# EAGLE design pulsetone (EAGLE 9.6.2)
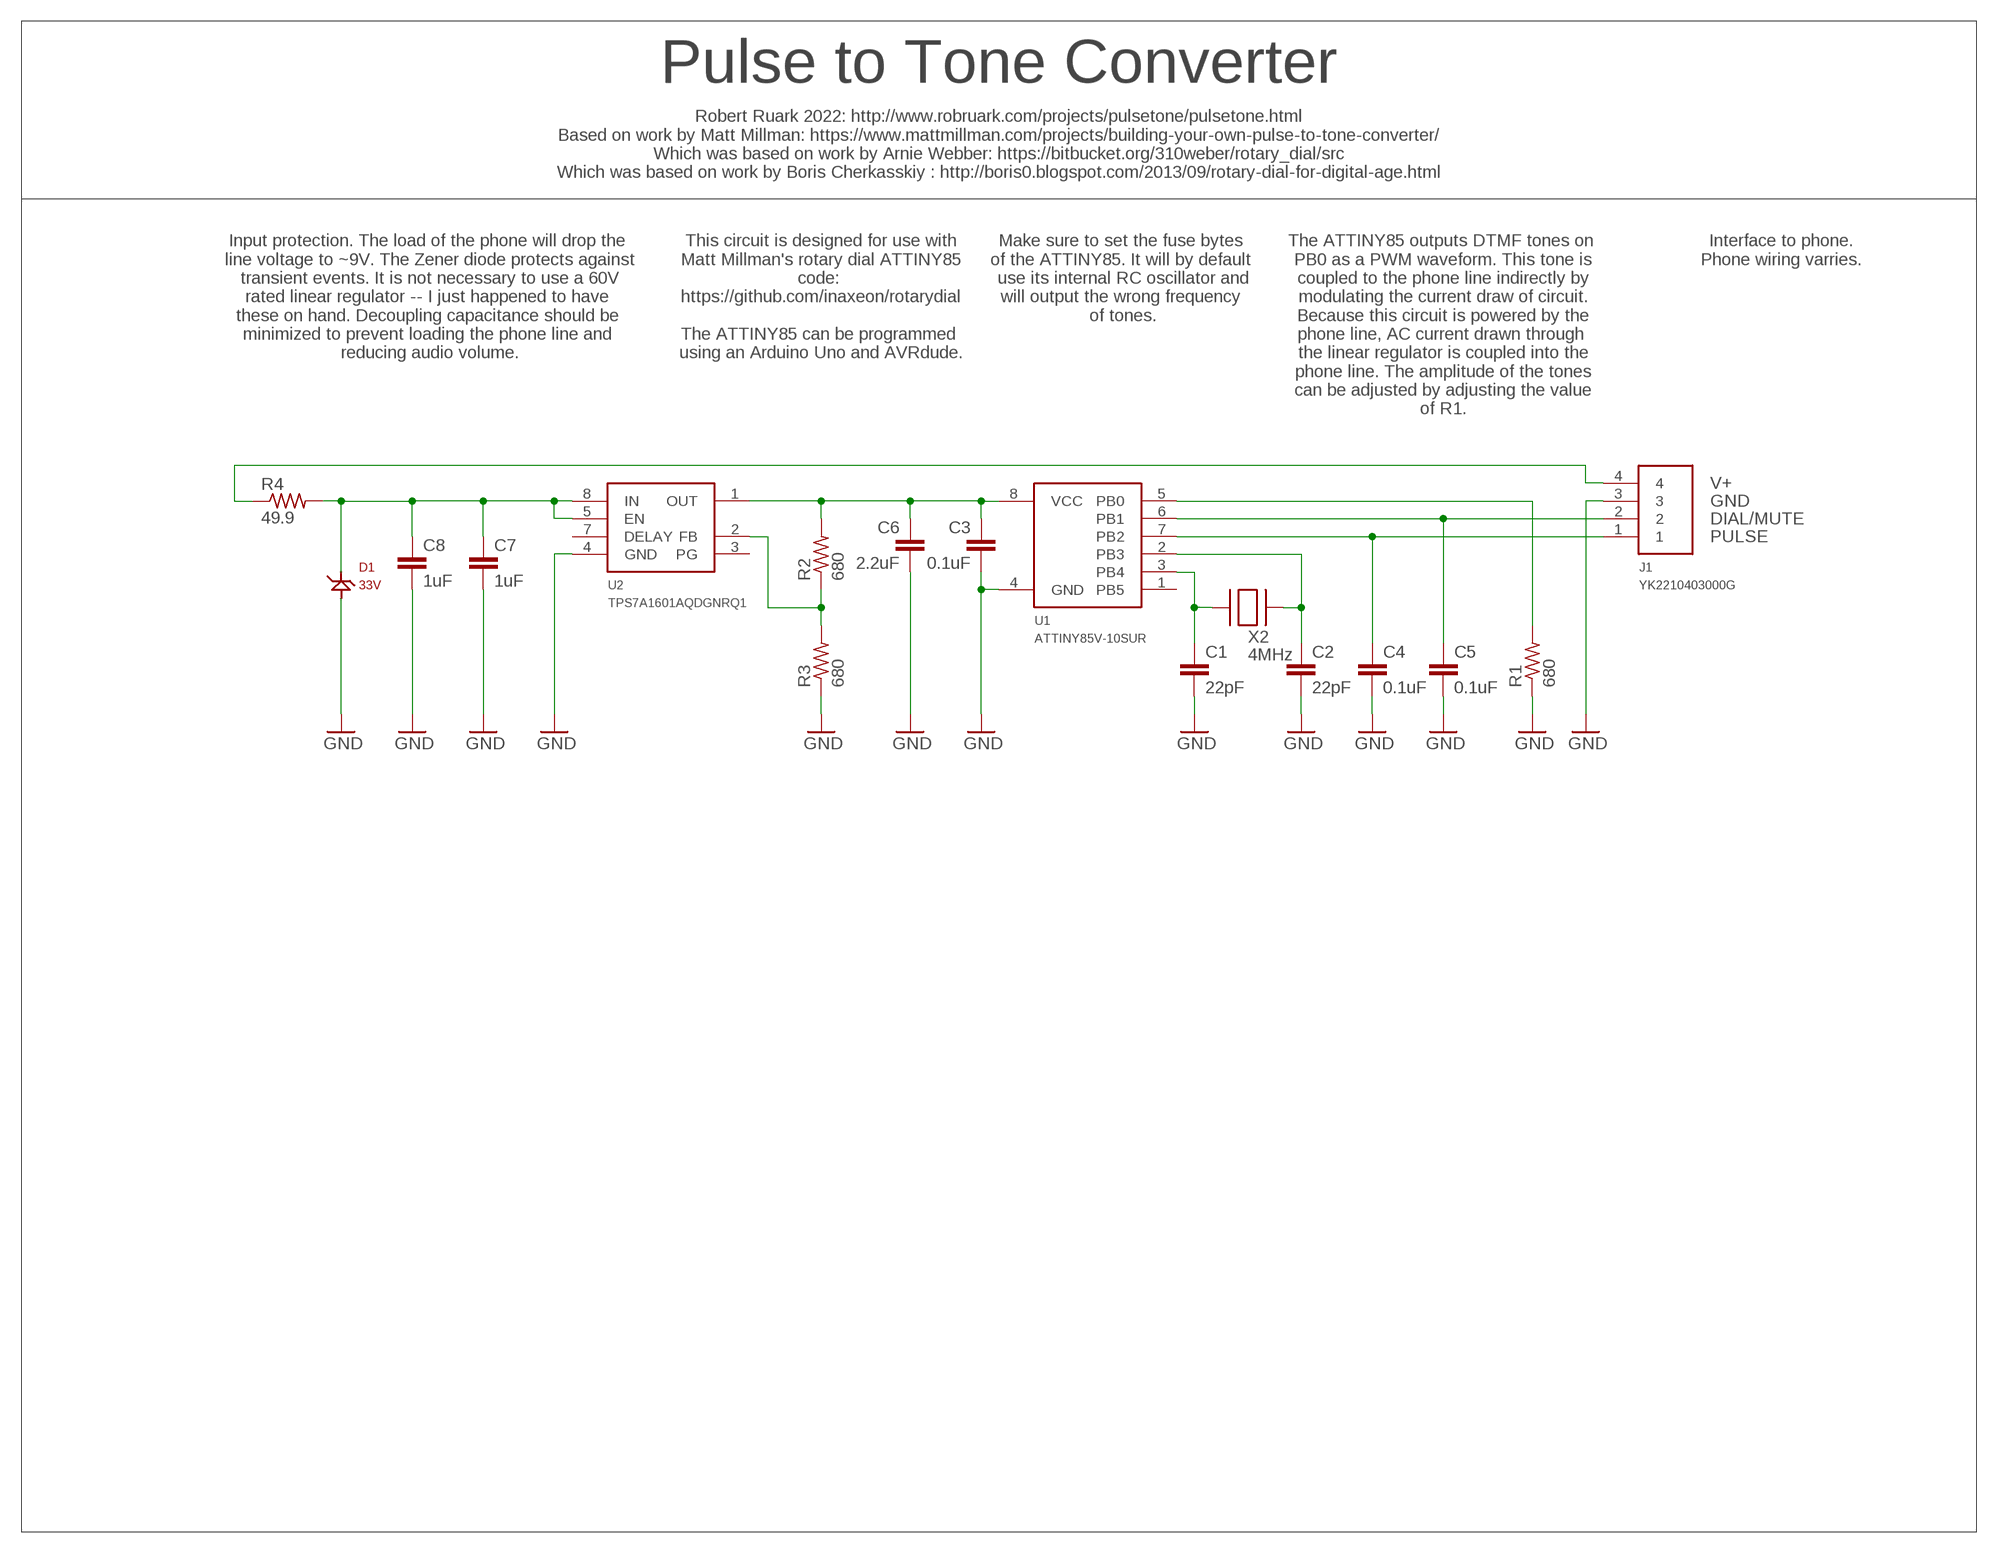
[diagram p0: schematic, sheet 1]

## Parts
C1  22pF  0603_CAPACITOR  [0603]
C2  22pF  0603_CAPACITOR  [0603]
C3  0.1uF  0603_CAPACITOR  [0603]
C4  0.1uF  0603_CAPACITOR  [0603]
C5  0.1uF  0603_CAPACITOR  [0603]
C6  2.2uF  0805_CAPACITOR  [0805]
C7  1uF  1206_CAPACITOR  [1206]
C8  1uF  1206_CAPACITOR  [1206]
D1  33V  1SMA5937BT3GDO-  [DO-214AC]
J1  YK2210403000G  [YK2210403000G]
R1  680  0603_RESISTOR  [0603]
R2  680  0603_RESISTOR  [0603]
R3  680  0603_RESISTOR  [0603]
R4  49.9  1206_RESISTOR  [1206]
U1  ATTINY85V-10SUR  [SOIC8]
U2  TPS7A1601AQDGNRQ1  [MSOP-8]
X2  4MHz  ABLS-4.000MHZ-B2-T  [HC-49/US]

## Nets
GND: C1.2 C2.2 C3.2 C4.2 C5.2 C6.2 C7.2 C8.2 D1.A J1.3 R1.1 R3.1 U1.4(GND) U2.4(GND)
N$1: C1.1 U1.3(PB4) X2.P$1
N$2: C2.1 U1.2(PB3) X2.P$2
N$3: C4.1 J1.1 U1.7(PB2)
N$4: C5.1 J1.2 U1.6(PB1)
N$5: R1.2 U1.5(PB0)
N$7: J1.4 R4.1
N$8: R2.1 R3.2 U2.2(FB)
N$10: C7.1 C8.1 D1.C(K) R4.2 U2.5(EN) U2.8(IN)
VCC: C3.1 C6.1 R2.2 U1.8(VCC) U2.1(OUT)
Unconnected: U1.1(PB5) U2.3(PG) U2.7(DELAY)

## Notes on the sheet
- Pulse to Tone Converter
- Robert Ruark 2022: http://www.robruark.com/projects/pulsetone/pulsetone.html
  Based on work by Matt Millman: https://www.mattmillman.com/projects/building-your-own-pulse-to-tone-converter/
  Which was based on work by Arnie Webber: https://bitbucket.org/310weber/rotary_dial/src
  Which was based on work by Boris Cherkasskiy : http://boris0.blogspot.com/2013/09/rotary-dial-for-digital-age.html
- Input protection. The load of the phone will drop the 
  line voltage to ~9V. The Zener diode protects against
  transient events. It is not necessary to use a 60V
  rated linear regulator -- I just happened to have 
  these on hand. Decoupling capacitance should be 
  minimized to prevent loading the phone line and 
  reducing audio volume.
- This circuit is designed for use with
  Matt Millman's rotary dial ATTINY85
  code: 
  https://github.com/inaxeon/rotarydial
  
  The ATTINY85 can be programmed 
  using an Arduino Uno and AVRdude.
- Make sure to set the fuse bytes 
  of the ATTINY85. It will by default 
  use its internal RC oscillator and
  will output the wrong frequency 
  of tones.
- The ATTINY85 outputs DTMF tones on 
  PB0 as a PWM waveform. This tone is
  coupled to the phone line indirectly by
  modulating the current draw of circuit.
  Because this circuit is powered by the
  phone line, AC current drawn through 
  the linear regulator is coupled into the
  phone line. The amplitude of the tones
  can be adjusted by adjusting the value
  of R1.
- Interface to phone.
  Phone wiring varries.
- V+
- GND
- DIAL/MUTE
- PULSE

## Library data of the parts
C1-C5 = ruark2:0603_CAPACITOR: 0603 Capacitor -- WARNING: NO DEFINED VALUE OR PART NUMBER; VALUE: sel
C6 = ruark2:0805_CAPACITOR: NO DEFINED PN
C7 C8 = ruark2:1206_CAPACITOR: NO DEFINED PN; VALUE: sel
D1 = ruark2:1SMA5937BT3G: Zener Diode 33 V 1.5 W ±5% Surface Mount SMA
J1 = ruark2:YK2210403000G: 4 Circuit 0.250" (6.35mm) Barrier Block Connector Screws with Captive Plate; PARTNO: YK2210403000G-ND
R1-R3 = ruark2:0603_RESISTOR: 0603 Resistor -- WARNING: NO DEFINED PART NUMBER OR VALUE; VALUE: sel
R4 = ruark2:1206_RESISTOR: NO DEFINED PN; VALUE: sel
U1 = ruark2:ATTINY85V-10SUR: AVR AVR® ATtiny, Functional Safety (FuSa) Microcontroller IC 8-Bit 10MHz 8KB (4K x 16) FLASH 8-SOIC; PARTNO: ATTINY85V-10SURCT-ND
U2 = ruark2:TPS7A1601AQDGNRQ1: Linear Voltage Regulator IC Positive Adjustable 60V 1 Output 100mA 8-HVSSOP
X2 = ruark2:ABLS-4.000MHZ-B2-T: 4 MHz ±20ppm Crystal 18pF 180 Ohms HC-49/US; PARTNO: 535-9085-1-ND

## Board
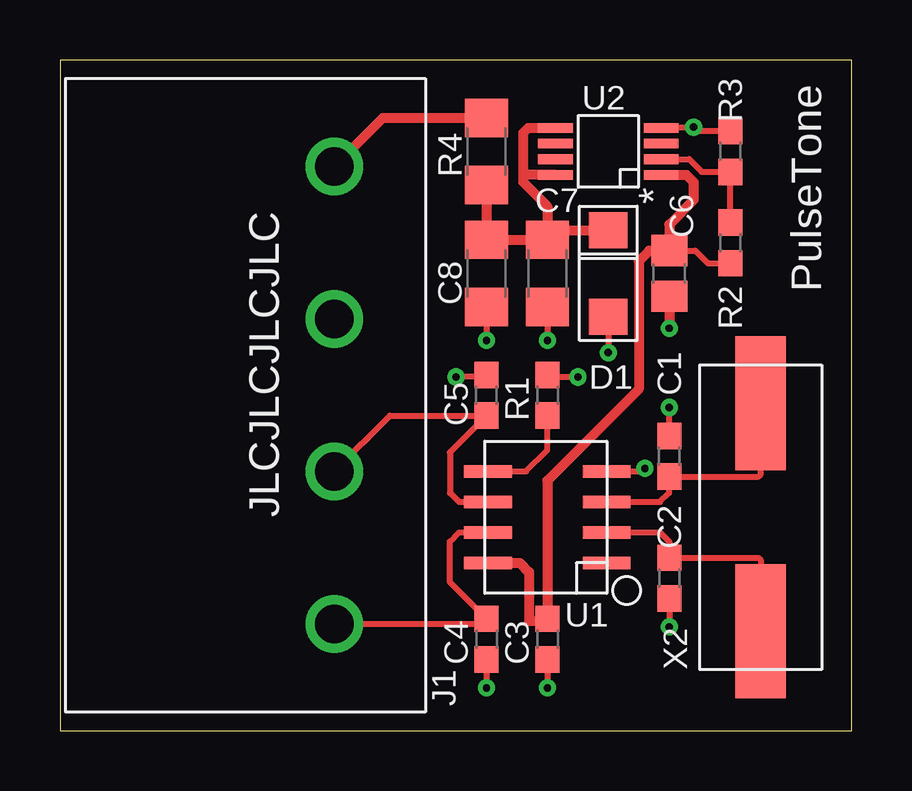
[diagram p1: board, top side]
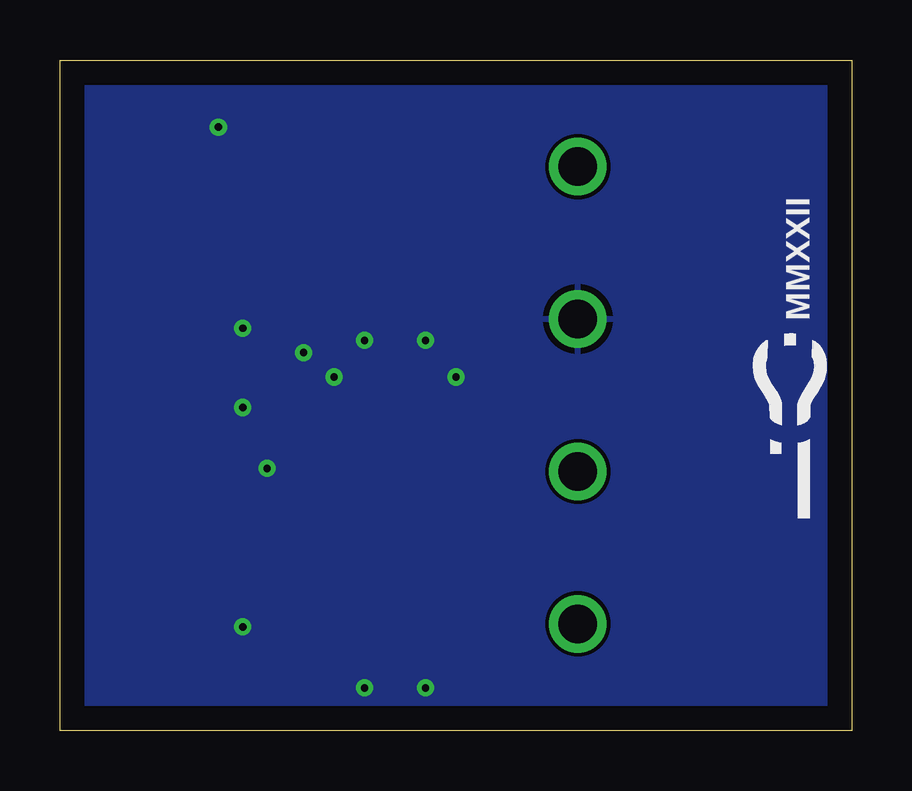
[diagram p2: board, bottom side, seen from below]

Size 33.02 x 27.94 mm. Coordinates in mm from the lower left corner, seen from the top.
Outline: 0,0 33.02,0 33.02,27.94 0,27.94 0,0
Copper layers (1*16): Top 0.035mm / dielectric 1.5mm / Bottom 0.035mm
Design rules "default": minimum track width 6mil, minimum drill 0.35mm, track to track 6mil, track to pad 6mil, pad to pad 6mil, via to via 6mil, smd to smd 6mil, copper to edge 40mil, drill to drill 6mil, minimum pad ring 10mil, minimum via ring 8mil, stop-mask expansion 4mil, vias tented up to drill 0mil, thermal gap 10mil

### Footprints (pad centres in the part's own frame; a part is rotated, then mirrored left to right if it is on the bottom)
0603 = smd 1.1 x 1: 1 -0.85,0; 2 0.85,0
0805 = smd 1.3 x 1.5: 1 -0.95,0; 2 0.95,0
1206 = smd 1.6 x 1.8: 1 -1.4,0; 2 1.4,0
DO-214AC = smd 1.5 x 1.6: A -1.8,0; C 1.8,0
YK2210403000G = drill 1.6: 1 -9.525,0; 2 -3.175,0; 3 3.175,0; 4 9.525,0
SOIC8 = smd 1.981 x 0.533: 1 -2.477,1.905; 2 -2.477,0.635; 3 -2.477,-0.635; 4 -2.477,-1.905; 5 2.477,-1.905; 6 2.477,-0.635; 7 2.477,0.635; 8 2.477,1.905
MSOP-8 = smd 1.45 x 0.4: 1 -2.2,0.975; 2 -2.2,0.325; 3 -2.2,-0.325; 4 -2.2,-0.975; 5 2.2,-0.975; 6 2.2,-0.325; 7 2.2,0.325; 8 2.2,0.975
HC-49/US = smd 5.588 x 2.108: P$1 4.75,0; P$2 -4.75,0

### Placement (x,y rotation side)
C1  25.4,11.43 90 top
C2  25.4,6.35 270 top
C3  20.32,3.81 270 top
C4  17.78,3.81 270 top
C5  17.78,13.97 90 top
C6  25.4,19.05 270 top
C7  20.32,19.05 270 top
C8  17.78,19.05 270 top
D1  22.86,19.05 90 top
J1  11.43,13.97 90 top
R1  20.32,13.97 270 top
R2  27.94,20.32 270 top
R3  27.94,24.13 270 top
R4  17.78,24.13 270 top
U1  20.32,8.89 180 top
U2  22.86,24.13 180 top
X2  29.21,8.89 90 top

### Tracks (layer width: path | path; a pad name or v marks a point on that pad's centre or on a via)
GND  (via drill 0.3)
  Top 0.254: C4.2 v17.78,1.78 | C3.2 v20.32,1.78 | C2.2 v25.4,4.32 | C1.2 v25.4,13.46 | D1.A v22.86,15.75 | R1.1 20.41,14.73 v21.59,14.73 | C5.2 17.69,14.73 v16.51,14.73 | C8.2 v17.78,16.26 | C7.2 v20.32,16.26 | U1.4 24.26,10.79 v24.38,10.92 | U2.4 25.1,25.15 v26.42,25.15 26.58,24.98 R3.1
  Top 0.406: C6.2 v25.4,16.76
  pour Bottom: 0,0 33.02,0 33.02,27.94 0,27.94
N$1
  Top 0.254: X2.P$1 29.21,10.67 29.12,10.58 C1.1 25.4,9.91 25.02,9.53 U1.3
N$2
  Top 0.254: U1.2 25.02,8.26 25.4,7.87 C2.1 29.12,7.2 29.21,7.11 X2.P$2
N$3
  Top 0.254: U1.7 16.64,8.26 16.26,7.87 16.26,6.18 C4.1 17.57,4.45 J1.1
N$4
  Top 0.254: U1.6 16.64,9.53 16.26,9.91 16.26,11.6 C5.1 13.76,13.12 J1.2
N$5
  Top 0.254: U1.5 19.43,10.79 20.32,11.68 R1.2
N$7
  Top 0.406: J1.4 13.46,25.53 R4.1
N$8
  Top 0.254: U2.2 26.23,23.8 26.76,23.28 R3.2 R2.1
N$10
  Top 0.254: C7.1 20.26,20.51 20.2,20.45 | D1.C 22.46,20.45
  Top 0.406: R4.2 C8.1 C7.1 | U2.5 19.52,25.11 19.3,24.89 19.3,23.11 | C7.1 20.32,21.84 19.3,22.86 19.3,23.11 | U2.8 19.34,23.16 19.3,23.11 | C7.1 20.72,20.85 D1.C
VCC
  Top 0.254: C6.1 26.48,20 27.01,19.47 R2.2
  Top 0.406: U2.1 26.12,23.16 26.42,22.86 26.42,22.1 25.4,21.08 C6.1 24.57,20 24.13,19.56 24.13,14.22 20.32,10.41 C3.1 20.23,4.57 19.56,4.57 19.56,6.6 19.18,6.99 U1.8

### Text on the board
bPlace: MMXXII
tNames: PulseTone | JLCJLCJLCJLC
bStop: 045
